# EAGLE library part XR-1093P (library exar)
EQUALIZER DISPLAY/FILTER/MULTIPLEXER
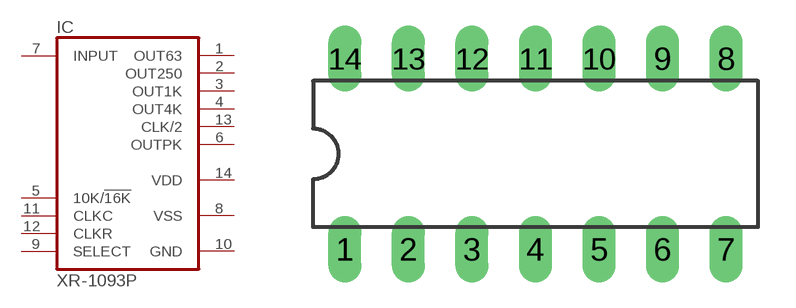
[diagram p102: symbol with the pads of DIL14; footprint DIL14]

Designator prefix IC

## XR-1093P (OC_FARNELL: unknown; OC_NEWARK: unknown)  [DIL14]
1  OUT63  out
2  OUT250  out
3  OUT1K  out
4  OUT4K  out
5  10K/!16K  in
6  OUTPK  out
7  INPUT  in
8  VSS  pwr
9  SELECT  in
10  GND  pwr
11  CLKC  in
12  CLKR  in
13  CLK/2  out
14  VDD  pwr

## Footprint DIL14 (pad centres in mm)
Dual In Line Package
drill 0.813 long: 1 -7.62,-3.81; 2 -5.08,-3.81; 3 -2.54,-3.81; 4 0,-3.81; 5 2.54,-3.81; 6 5.08,-3.81; 7 7.62,-3.81; 8 7.62,3.81; 9 5.08,3.81; 10 2.54,3.81; 11 0,3.81; 12 -2.54,3.81; 13 -5.08,3.81; 14 -7.62,3.81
